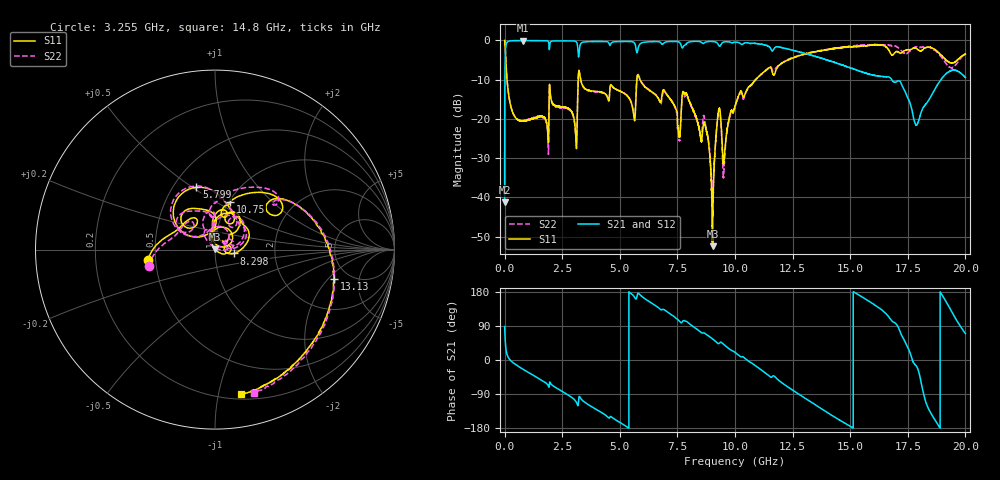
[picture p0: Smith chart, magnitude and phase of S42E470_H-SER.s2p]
! Created Wed Nov 25 22:17:46 2020
# khz S ma R 50
! 2 Port Network Data from SP1.SP block
! freq  magS11  angS11  magS21  angS21  magS12  angS12  magS22  angS22
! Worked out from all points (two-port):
!   20001 points, 300 kHz to 20 GHz, reference 50 ohm
!   highest |S21| = -0.05 dB at 806.3 MHz (marker M1); lowest = -41.3 dB at 300 kHz (marker M2)
!   |S21| within 3 dB of the highest: 34.56 MHz to 3.19 GHz (3.156 GHz wide, 196 % of centre); 5.756 GHz to 12.85 GHz (7.09 GHz wide, 76.2 % of centre)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
!   lowest |S11| = -52.4 dB at 9.028 GHz (marker M3), VSWR 1.00, Z = 50 + j0.235 ohm
!   |S11| at or under -10 dB: 105.7 MHz to 3.195 GHz (3.089 GHz wide, 187 % of centre); 3.302 GHz to 5.74 GHz (2.439 GHz wide, 53.9 % of centre); 5.878 GHz to 10.89 GHz (5.014 GHz wide, 59.8 % of centre)
!   |S22| runs from -39.9 to 0.0 dB; largest |S21 - S12| = 0.012
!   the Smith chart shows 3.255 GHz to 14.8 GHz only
!   S11 on the Smith chart (normalised r, x): 3.255 GHz: 0.45, -0.06; 5.799 GHz: 0.65, +0.52; 8.298 GHz: 1.24, -0.05; 10.75 GHz: 1.02, +0.58; 13.13 GHz: 3.80, -2.33; 14.8 GHz: 0.24, -1.17
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300  0.9968 -0.7  0.008658 88.2  0.008698 89.0  0.9968 -0.7
121300  0.2807 -78.3  0.9589 11.8  0.9588 11.8  0.282 -78.2
806300  0.09401 -115.6  0.9946 -24.7  0.9933 -24.6  0.09497 -115.4
3060300  0.07877 169.1  0.9779 -106.5  0.9776 -106.5  0.07737 179.6
3255300  0.3778 -171.4  0.8101 -96.5  0.8092 -96.6  0.3787 -165.6
3334300  0.2907 167.6  0.9296 -103.7  0.9281 -103.7  0.2886 174.2
5592300  0.1184 93.1  0.9528 169.4  0.9526 169.4  0.1243 99.6
5799300  0.3623 106.7  0.8021 176.3  0.8019 176.3  0.3716 107.8
6667300  0.1843 56.0  0.9655 138.4  0.9648 138.4  0.1839 49.5
8298300  0.1081 -11.4  0.9724 83.4  0.9709 83.6  0.1041 4.1
9028300  0.002391 78.8  0.9708 55.4  0.9713 55.3  0.01143 68.4
9282300  0.1254 79.4  0.8761 43.3  0.8755 43.2  0.1256 89.1
9526300  0.03058 80.5  0.9566 40.2  0.9579 40.2  0.02317 110.7
1.00003e7  0.1457 95.7  0.9512 20.1  0.9514 20.1  0.1411 116.9
1.07483e7  0.2778 72.1  0.9185 -8.8  0.9175 -8.8  0.28 85.9
1.31273e7  0.6828 -13.9  0.6721 -104.2  0.6713 -104.0  0.6859 -14.0
1.33343e7  0.7021 -21.9  0.6441 -112.3  0.6497 -112.2  0.7071 -22.0
1.48013e7  0.8163 -79.7  0.4689 -167.6  0.4692 -168.0  0.8297 -74.9
1.66673e7  0.7604 -150.7  0.3442 114.5  0.3358 115.1  0.8702 -146.8
1.78743e7  0.7921 -178.5  0.08334 -16.1  0.08524 -17.2  0.8245 -174.2
1.91153e7  0.5819 132.9  0.3655 158.7  0.3656 158.2  0.53 138.8
2e7  0.6697 130.4  0.3373 69.8  0.3402 70.7  0.6777 136.7
